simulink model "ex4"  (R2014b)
settings: Solver=ode45  StartTime=0.0  StopTime=10.0  RelTol=1e-3

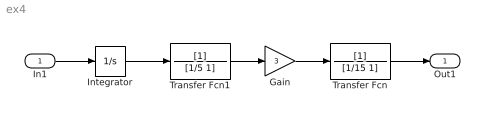
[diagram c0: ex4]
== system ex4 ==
  In1 : Inport
  Gain : Gain  Gain=3
  Integrator : Integrator
  Transfer Fcn : TransferFcn  Denominator=[1/15 1]
  Transfer Fcn1 : TransferFcn  Denominator=[1/5 1]
  Out1 : Outport
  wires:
  Transfer Fcn/1 -> Out1/1
  Transfer Fcn1/1 -> Gain/1
  Gain/1 -> Transfer Fcn/1
  In1/1 -> Integrator/1
  Integrator/1 -> Transfer Fcn1/1
